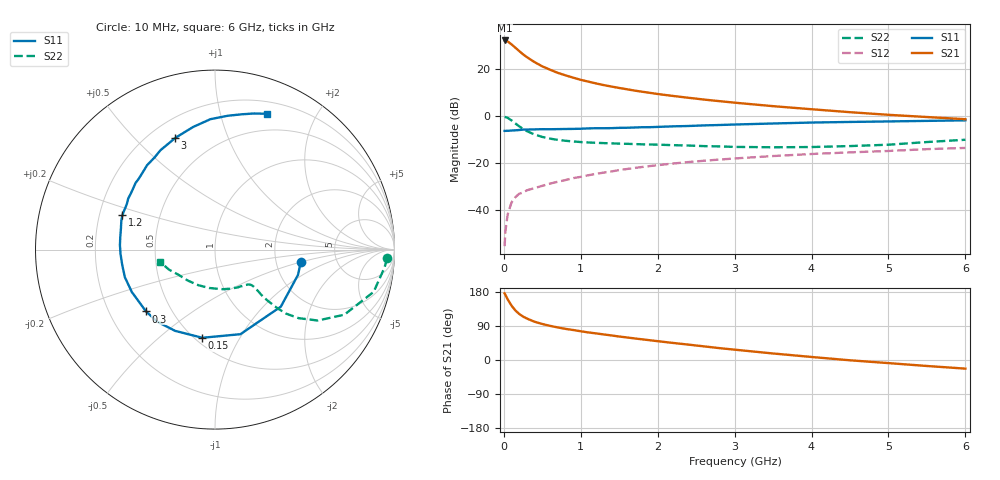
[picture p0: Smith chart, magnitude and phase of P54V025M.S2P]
! SIEMENS Small Signal Semiconductors
! BFP183
! Si NPN RF Bipolar Junction Transistor in SOT143
! VCE = 4 V  IC = 25 mA
! Common Emitter S-Parameters:  March  1996
# GHz  S  MA  R  50
!  f  S11  S21  S12  S22
! GHz  MAG  ANG  MAG  ANG  MAG  ANG  MAG  ANG
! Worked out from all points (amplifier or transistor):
!   36 points, 10 MHz to 6 GHz, reference 50 ohm
!   highest |S21| = 32.2 dB at 10 MHz (marker M1)
!   |S21| within 3 dB of that: start of sweep to 147.3 MHz
!   unconditionally stable (mu >= 1): 734.3 MHz to 5.603 GHz
!   at 250 MHz: K = 0.53, MSG = 29.4 dB, |S12| = -32.5 dB
!   at 1.4 GHz: K = 1.15, MAG = 15.7 dB, |S12| = -23.6 dB
!   at 6 GHz: K = 0.96, MSG = 6.1 dB, |S12| = -13.6 dB
!   S11 on the Smith chart (normalised r, x): 10 MHz: 2.77, -0.49; 150 MHz: 0.54, -0.71; 300 MHz: 0.36, -0.34; 1.2 GHz: 0.30, +0.17; 3 GHz: 0.30, +0.66; 6 GHz: 0.32, +1.41
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0.01  0.4834 -8.0  40.63 175.8  0.0017 83.9  0.96 -2.9
0.02  0.4834 -17.0  40.55 172.0  0.0035 81.0  0.95 -6.0
0.05  0.4854 -40.9  38.8 159.9  0.0081 76.4  0.915 -14.9
0.1  0.4921 -73.3  33.52 143.5  0.0145 63.6  0.807 -26.7
0.15  0.4963 -98.2  28.51 130.7  0.0188 57.5  0.6959 -34.6
0.2  0.5042 -116.1  24.15 121.5  0.0222 53.7  0.6034 -39.3
0.25  0.5148 -128.6  20.57 114.5  0.0236 51.4  0.5334 -42.0
0.3  0.5161 -138.1  17.93 109.4  0.0263 50.5  0.4774 -43.2
0.4  0.5202 -153.0  14.03 100.9  0.0293 50.7  0.4042 -44.2
0.5  0.5252 -163.0  11.41 95.0  0.0327 51.1  0.3594 -44.3
0.6  0.5239 -170.5  9.702 90.1  0.0365 52.4  0.3309 -43.9
0.7  0.527 -177.4  8.309 86.0  0.0399 53.7  0.3112 -43.8
0.8  0.5303 177.2  7.359 82.2  0.0434 54.3  0.2979 -43.8
1.1  0.5458 163.0  5.391 72.7  0.055 55.0  0.2737 -45.3
1.2  0.551 159.5  4.938 70.2  0.0588 55.1  0.2694 -46.2
1.7  0.5706 142.6  3.482 56.9  0.0786 53.5  0.2535 -53.3
2.2  0.6037 128.8  2.677 45.0  0.0976 49.8  0.2398 -63.0
3  0.6602 109.7  1.926 27.3  0.1251 42.8  0.2205 -83.5
3.5  0.6941 100.1  1.623 17.2  0.1408 38.2  0.2163 -98.7
4.5  0.7489 84.6  1.208 -0.8  0.1687 29.0  0.2296 -131.3
5.5  0.7889 74.0  0.953 -15.8  0.1975 21.1  0.2798 -156.5
6  0.8105 69.0  0.857 -22.8  0.2096 16.5  0.313 -167.3
